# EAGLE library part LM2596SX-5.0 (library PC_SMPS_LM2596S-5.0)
Voltage Regulator
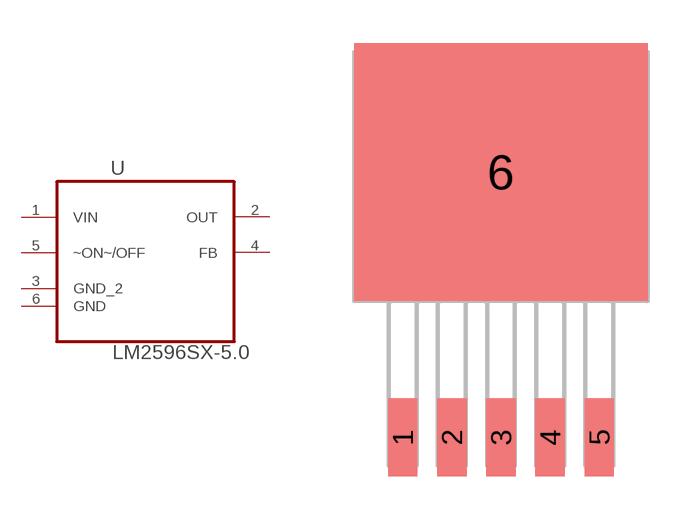
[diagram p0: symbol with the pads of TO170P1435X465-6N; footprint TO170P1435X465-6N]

Designator prefix U

## LM2596SX-5.0 (Availability: Unavailable; Description: Ic, Step-Down Volt Regulator 5v To-220-5, Full Reel; MF: Texas Instruments; MP: LM2596SX-5.0; Package: TO-263-5 Texas Instruments; Price: None)  [TO170P1435X465-6N]
1  VIN  in
2  OUT  out
3  GND_2  pas
4  FB
5  ~ON~/OFF  pas
6  GND  pas

## Footprint TO170P1435X465-6N (pad centres in mm)
smd 1.016 x 2.692: 1 -3.404,-9.042; 2 -1.702,-9.042; 3 0,-9.042; 4 1.702,-9.042; 5 3.404,-9.042
smd 10.16 x 8.941: 6 0,0.152

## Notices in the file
This work is licensed under a Creative Commons Attribution-ShareAlike 4.0 International License (CC BY-SA) with Design Exception 1.0
